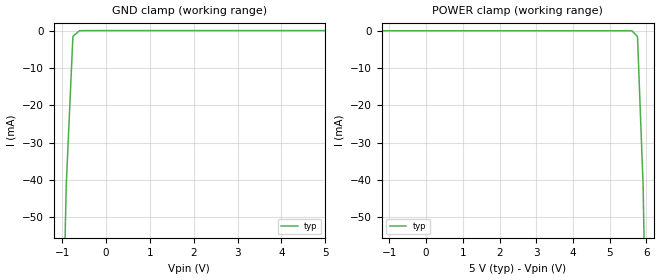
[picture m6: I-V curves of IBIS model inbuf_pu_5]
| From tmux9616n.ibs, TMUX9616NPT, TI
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| inbuf_pu_5
[Model]   inbuf_pu_5
Model_type   Input
Vinl = 1.5
Vinh = 3
|   typ   min   max
C_comp   1.008417e-12   NA   NA
[Voltage Range]   5   NA   NA
[Temperature Range]   27   NA   NA
[Power Clamp Reference]   5   NA   NA
[GND Clamp Reference]   0   NA   NA
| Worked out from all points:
|   GND clamp passes 1 mA (typ) near -0.70 V on its own axis
[GND Clamp]
|   Voltage   I(typ)   I(min)   I(max)
-10V      -5.956A    NA         NA
-1.061V   -120.6mA   NA         NA
-909.1mV  -41.17mA   NA         NA
-757.6mV  -1.548mA   NA         NA
-606.1mV  -26.51uA   NA         NA
5V        36.69pA    NA         NA
[POWER Clamp]
|   Voltage   I(typ)   I(min)   I(max)
-5V       49uA       NA         NA
5.606V    -26.51uA   NA         NA
5.758V    -1.548mA   NA         NA
5.909V    -41.17mA   NA         NA
6.061V    -120.6mA   NA         NA
10V       -2.663A    NA         NA
